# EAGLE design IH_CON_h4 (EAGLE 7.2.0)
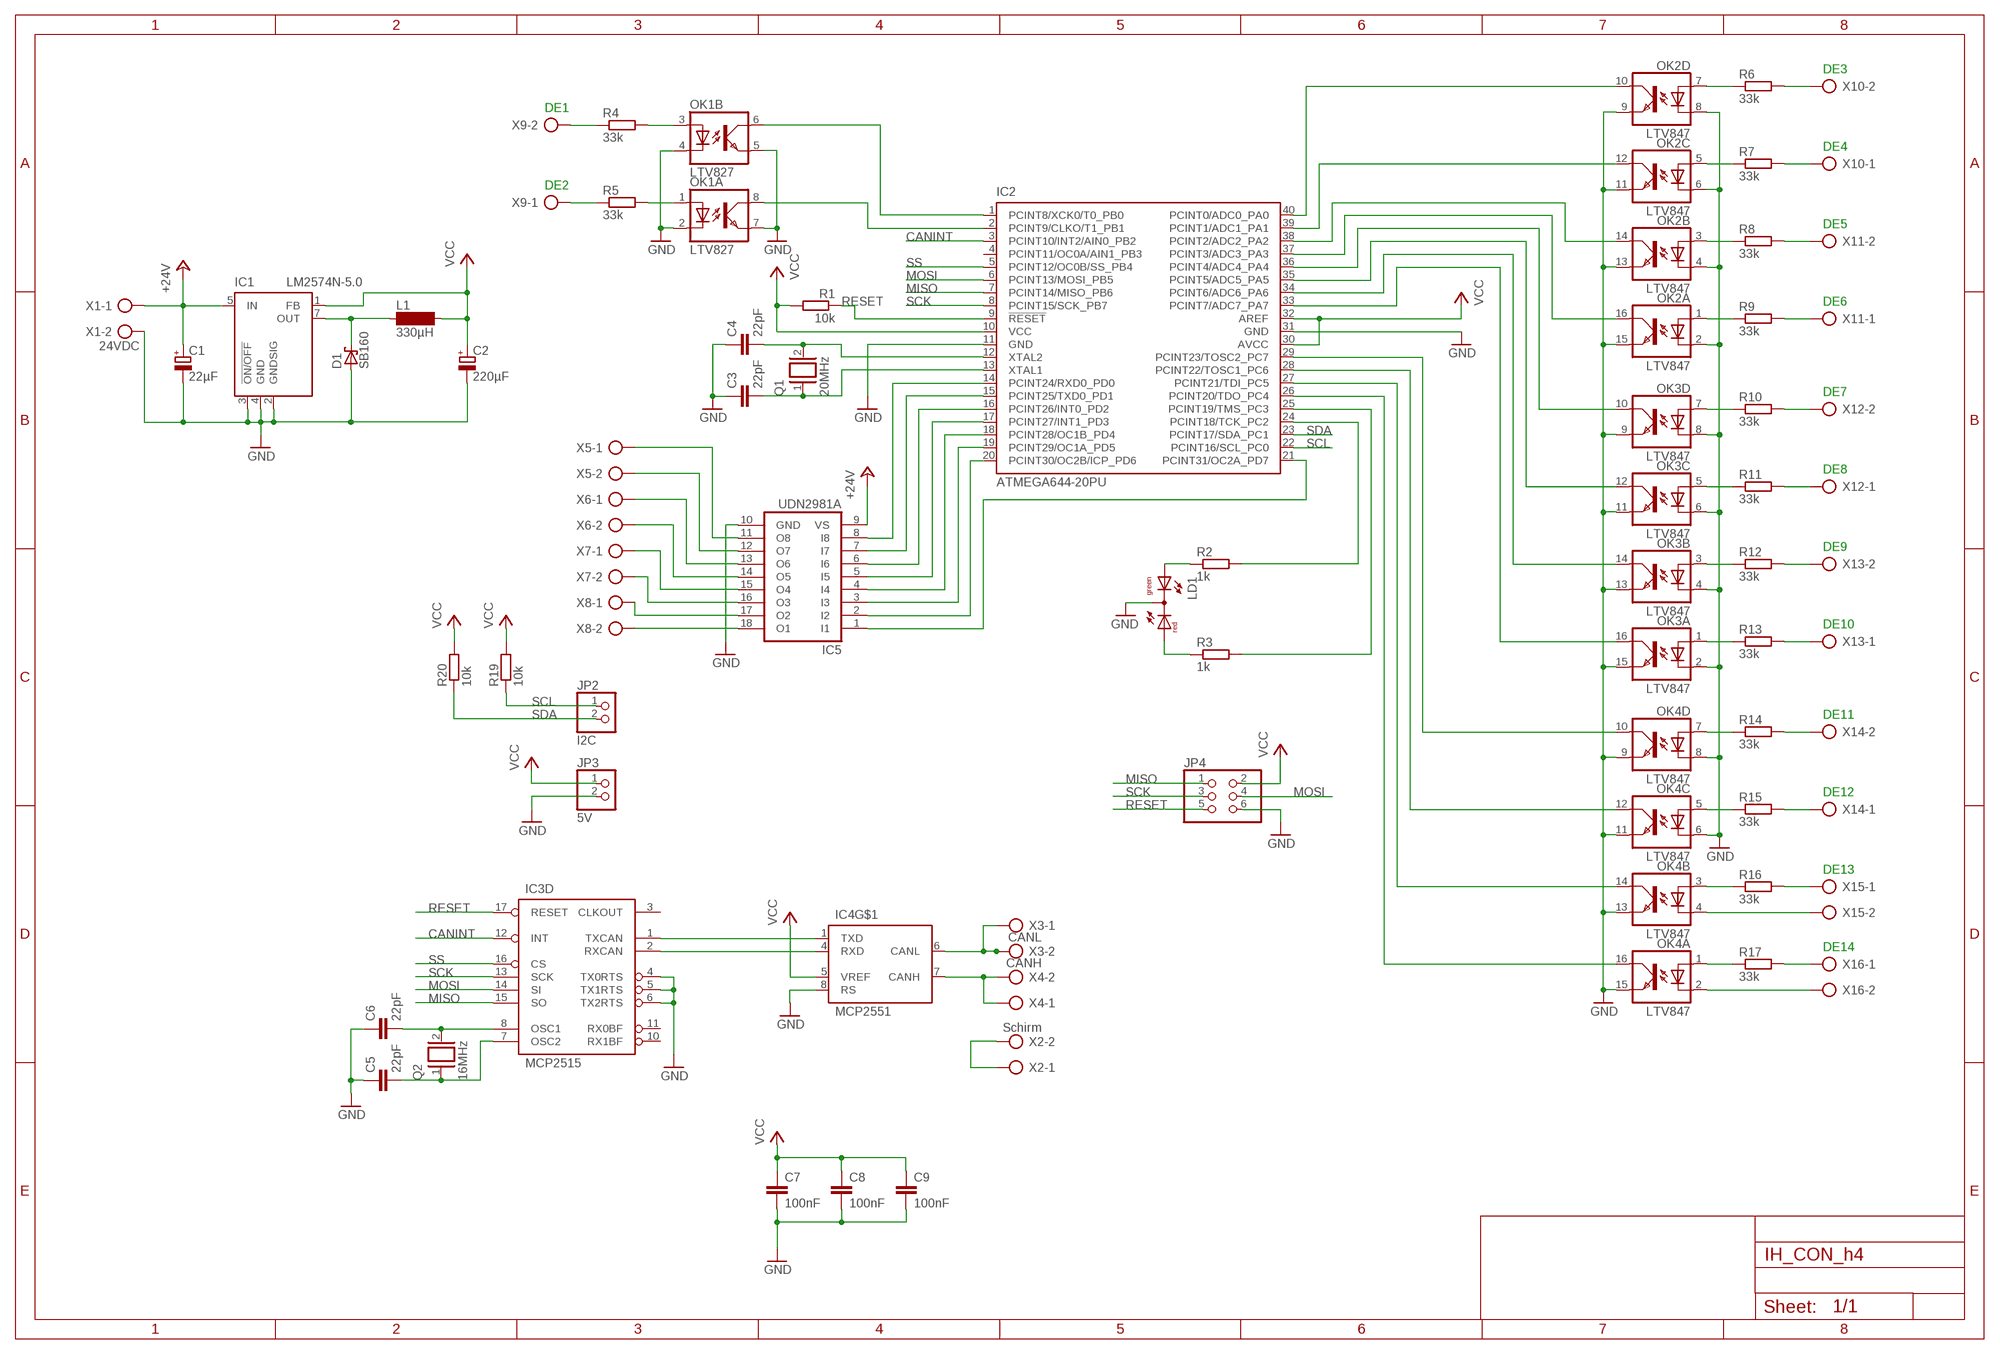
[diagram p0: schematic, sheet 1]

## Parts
C1  22µF  CPOL-EUE2-5  [E2-5]
C2  220µF  CPOL-EUE3.5-8  [E3,5-8]
C3  22pF  C-EUC0805  [C0805]
C4  22pF  C-EUC0805  [C0805]
C5  22pF  C-EUC0805  [C0805]
C6  22pF  C-EUC0805  [C0805]
C7  100nF  C-EUC0805  [C0805]
C8  100nF  C-EUC0805  [C0805]
C9  100nF  C-EUC0805  [C0805]
D1  SB160  SCHOTTKY-DIODEF126Z12  [F126Z12]
IC1  LM2574N-5.0  [DIL08]
IC2  ATMEGA644-20PU  [DIL40]
IC3  MCP2515  MCP2515P  [DIL18]
IC4  MCP2551  MCP2551DIL8  [DIL08]
IC5  UDN2981A  [DIL18]
JP2  I2C  PINHD-1X2  [1X02]
JP3  5V  PINHD-1X2  [1X02]
JP4  PINHD-2X3  [2X03]
L1  330µH  SD12-1000  [SD12_1000]
LD1  DUOLED-RG-C  [DUOLED-C-5MM]
OK1  LTV827  PC827  [DIL08]
OK2  LTV847  PC847  [DIL16]
OK3  LTV847  PC847  [DIL16]
OK4  LTV847  PC847  [DIL16]
Q1  20MHz  XTAL/S  [QS]
Q2  16MHz  XTAL/S  [QS]
R1  10k  R-EU_M0805  [M0805]
R2  1k  R-EU_M0805  [M0805]
R3  1k  R-EU_M0805  [M0805]
R4  33k  R-EU_0207/2V  [0207/2V]
R5  33k  R-EU_0207/2V  [0207/2V]
R6  33k  R-EU_0207/2V  [0207/2V]
R7  33k  R-EU_0207/2V  [0207/2V]
R8  33k  R-EU_0207/2V  [0207/2V]
R9  33k  R-EU_0207/2V  [0207/2V]
R10  33k  R-EU_0207/2V  [0207/2V]
R11  33k  R-EU_0207/2V  [0207/2V]
R12  33k  R-EU_0207/2V  [0207/2V]
R13  33k  R-EU_0207/2V  [0207/2V]
R14  33k  R-EU_0207/2V  [0207/2V]
R15  33k  R-EU_0207/2V  [0207/2V]
R16  33k  R-EU_0207/2V  [0207/2V]
R17  33k  R-EU_0207/2V  [0207/2V]
R19  10k  R-EU_M0805  [M0805]
R20  10k  R-EU_M0805  [M0805]
X1  24VDC  AK300/2  [AK300/2]
X2  Schirm  AK300/2  [AK300/2]
X3  CANL  AK300/2  [AK300/2]
X4  CANH  AK300/2  [AK300/2]
X5  AK300/2  [AK300/2]
X6  AK300/2  [AK300/2]
X7  AK300/2  [AK300/2]
X8  AK300/2  [AK300/2]
X9  AK300/2  [AK300/2]
X10  AK300/2  [AK300/2]
X11  AK300/2  [AK300/2]
X12  AK300/2  [AK300/2]
X13  AK300/2  [AK300/2]
X14  AK300/2  [AK300/2]
X15  AK300/2  [AK300/2]
X16  AK300/2  [AK300/2]

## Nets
+24V: C1.+ IC1.5(IN) IC5.9(VS) X1.1
CANINT: IC2.3(PCINT10/INT2/AIN0_PB2) IC3.12(D:INT)
GND: C1.- C2.- C3.1 C4.1 C5.1 C6.1 C7.2 C8.2 C9.2 D1.A IC1.2(GNDSIG) IC1.3(!ON/OFF) IC1.4(GND) IC2.11(GND) IC2.31(GND) IC3.4(D:TX0RTS) IC3.5(D:TX1RTS) IC3.6(D:TX2RTS) IC4.8(RS) IC5.10(GND) JP3.2 JP4.6 LD1.C OK1.2(A:C) OK1.4(B:C) OK1.5(B:EMIT) OK1.7(A:EMIT) OK2.2(A:C) OK2.4(B:C) OK2.6(C:C) OK2.8(D:C) OK2.9(D:EMIT) OK2.11(C:EMIT) OK2.13(B:EMIT) OK2.15(A:EMIT) OK3.2(A:C) OK3.4(B:C) OK3.6(C:C) OK3.8(D:C) OK3.9(D:EMIT) OK3.11(C:EMIT) OK3.13(B:EMIT) OK3.15(A:EMIT) OK4.6(C:C) OK4.8(D:C) OK4.9(D:EMIT) OK4.11(C:EMIT) OK4.13(B:EMIT) OK4.15(A:EMIT) X1.2
MISO: IC2.7(PCINT14/MISO_PB6) IC3.15(D:SO) JP4.1
MOSI: IC2.6(PCINT13/MOSI_PB5) IC3.14(D:SI) JP4.4
N$1: IC3.1(D:TXCAN) IC4.1(TXD)
N$2: IC3.2(D:RXCAN) IC4.4(RXD)
N$3: C6.2 IC3.8(D:OSC1) Q2.2
N$4: C5.2 IC3.7(D:OSC2) Q2.1
N$5: IC2.14(PCINT24/RXD0_PD0) IC5.8(I8)
N$6: IC2.15(PCINT25/TXD0_PD1) IC5.7(I7)
N$7: C4.2 IC2.12(XTAL2) Q1.2
N$8: C3.2 IC2.13(XTAL1) Q1.1
N$9: IC2.21(PCINT31/OC2A_PD7) IC5.1(I1)
N$10: IC2.16(PCINT26/INT0_PD2) IC5.6(I6)
N$11: IC2.17(PCINT27/INT1_PD3) IC5.5(I5)
N$12: IC2.18(PCINT28/OC1B_PD4) IC5.4(I4)
N$13: IC2.19(PCINT29/OC1A_PD5) IC5.3(I3)
N$14: IC2.20(PCINT30/OC2B/ICP_PD6) IC5.2(I2)
N$16: IC4.6(CANL) X3.1 X3.2
N$17: IC4.7(CANH) X4.1 X4.2
N$18: IC5.18(O1) X8.2
N$19: IC5.17(O2) X8.1
N$20: IC5.16(O3) X7.2
N$21: IC5.15(O4) X7.1
N$22: IC5.14(O5) X6.2
N$23: IC5.13(O6) X6.1
N$24: IC5.12(O7) X5.2
N$25: IC5.11(O8) X5.1
N$26: IC2.25(PCINT19/TMS_PC3) R3.2
N$27: R6.2 X10.2
N$28: OK4.1(A:A) R17.1
N$29: OK4.3(B:A) R16.1
N$30: OK4.5(C:A) R15.1
N$31: OK4.7(D:A) R14.1
N$32: OK3.1(A:A) R13.1
N$33: IC2.24(PCINT18/TCK_PC2) R2.2
N$34: OK3.3(B:A) R12.1
N$35: OK3.5(C:A) R11.1
N$36: OK3.7(D:A) R10.1
N$37: OK2.1(A:A) R9.1
N$38: OK2.3(B:A) R8.1
N$39: OK2.5(C:A) R7.1
N$40: OK2.7(D:A) R6.1
N$41: R7.2 X10.1
N$42: LD1.AX(AG) R2.1
N$43: LD1.AR R3.1
N$45: R8.2 X11.2
N$46: R9.2 X11.1
N$47: R10.2 X12.2
N$48: R11.2 X12.1
N$49: R12.2 X13.2
N$50: R13.2 X13.1
N$51: R14.2 X14.2
N$52: R15.2 X14.1
N$53: R16.2 X15.1
N$54: X2.1 X2.2
N$55: R17.2 X16.1
N$56: OK4.2(A:C) X16.2
N$57: IC2.33(PCINT7/ADC7_PA7) OK3.16(A:COL)
N$58: IC2.34(PCINT6/ADC6_PA6) OK3.14(B:COL)
N$59: IC2.35(PCINT5/ADC5_PA5) OK3.12(C:COL)
N$60: IC2.36(PCINT4/ADC4_PA4) OK3.10(D:COL)
N$61: IC2.37(PCINT3/ADC3_PA3) OK2.16(A:COL)
N$62: IC2.38(PCINT2/ADC2_PA2) OK2.14(B:COL)
N$63: IC2.39(PCINT1/ADC1_PA1) OK2.12(C:COL)
N$64: IC2.40(PCINT0/ADC0_PA0) OK2.10(D:COL)
N$65: IC2.29(PCINT23/TOSC2_PC7) OK4.10(D:COL)
N$66: IC2.28(PCINT22/TOSC1_PC6) OK4.12(C:COL)
N$67: IC2.27(PCINT21/TDI_PC5) OK4.14(B:COL)
N$68: IC2.26(PCINT20/TDO_PC4) OK4.16(A:COL)
N$71: OK1.3(B:A) R4.2
N$72: R5.1 X9.1
N$73: R4.1 X9.2
N$74: IC2.2(PCINT9/CLKO/T1_PB1) OK1.8(A:COL)
N$75: IC2.1(PCINT8/XCK0/T0_PB0) OK1.6(B:COL)
N$76: D1.C IC1.7(OUT) L1.1
N$100: OK4.4(B:C) X15.2
OK1: OK1.1(A:A) R5.2
RESET: IC2.9(!RESET) IC3.17(D:RESET) JP4.5 R1.1
SCK: IC2.8(PCINT15/SCK_PB7) IC3.13(D:SCK) JP4.3
SCL: IC2.22(PCINT16/SCL_PC0) JP2.1 R19.1
SDA: IC2.23(PCINT17/SDA_PC1) JP2.2 R20.1
SS: IC2.5(PCINT12/OC0B/SS_PB4) IC3.16(D:CS)
VCC: C2.+ C7.1 C8.1 C9.1 IC1.1(FB) IC2.10(VCC) IC2.30(AVCC) IC2.32(AREF) IC4.5(VREF) JP3.1 JP4.2 L1.2 R1.2 R19.2 R20.2
Unconnected: IC2.4(PCINT11/OC0A/AIN1_PB3) IC3.3(D:CLKOUT) IC3.10(D:RX1BF) IC3.11(D:RX0BF)

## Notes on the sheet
- DE3
- DE1
- DE4
- DE2
- DE5
- DE6
- DE7
- DE8
- DE9
- DE10
- DE11
- DE12
- DE13
- DE14

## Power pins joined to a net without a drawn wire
GND: IC3.9(P:GND) IC4.2(GND)
VCC: IC3.18(P:VCC) IC4.3(VCC)

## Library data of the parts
C1 C2 = rcl:CPOL-EU: POLARIZED CAPACITOR, European symbol
C3-C9 = rcl:C-EU: CAPACITOR, European symbol
D1 = diode:SCHOTTKY-DIODE: Schottky Diode
IC1 = linear:LM2574?-*: SIMPLE SWITCHER 0.5A Step-Down Voltage Regulator Source: http://cache.national.com/ds/LM/LM2574.pdf
IC2 = atmel:ATMEGA644-*PU: 8-bit Microcontroller with 64K Bytes In-System Programmable Flash Auto generated by make-symbol-device-package-bsdl.ulp Rev. 34 Source: http://www.atmel.com/dyn/resources/prod_documents/doc2593.pdf; MPN: ATMEGA644-20PU; OC_FARNELL: 1288340; OC_NEWARK: 23M5060
IC3 = can:MCP2515: MC2515 Stand-Alone CAN Controller With SPI Interface, Microchip
IC4 = can:MCP2551: CAN Tranceiver Microchip
IC5 = uln-udn:UDN298*: DRIVER ARRAY Source: Allegro Microsystems Inc. / UDN2981-UDN2984.pdf
JP2 JP3 = pinhead:PINHD-1X2: PIN HEADER
JP4 = pinhead:PINHD-2X3: PIN HEADER
L1 = inductor-neosid:SD12: INDUCTOR; OC_FARNELL: unknown; OC_NEWARK: unknown
LD1 = led:DUOLED-RG-C: DUO LED 2 colors (red/green), 5 mm, round, common Cathode www.ligitek.com or other producers.
OK1 = optocoupler:PC827: SHARP OPTO COUPLER; OC_FARNELL: unknown; OC_NEWARK: unknown
OK2-OK4 = optocoupler:PC847: SHARP OPTO COUPLER; OC_FARNELL: 9707735; OC_NEWARK: unknown
Q1 Q2 = special:XTAL/S: CRYSTAL
R1 = rcl:R-EU_: RESISTOR, European symbol
R2-R17 R19 R20 = resistor:R-EU_: RESISTOR, European symbol
X1-X16 = con-ptr500:AK300/2: CONNECTOR; OC_FARNELL: unknown; OC_NEWARK: unknown

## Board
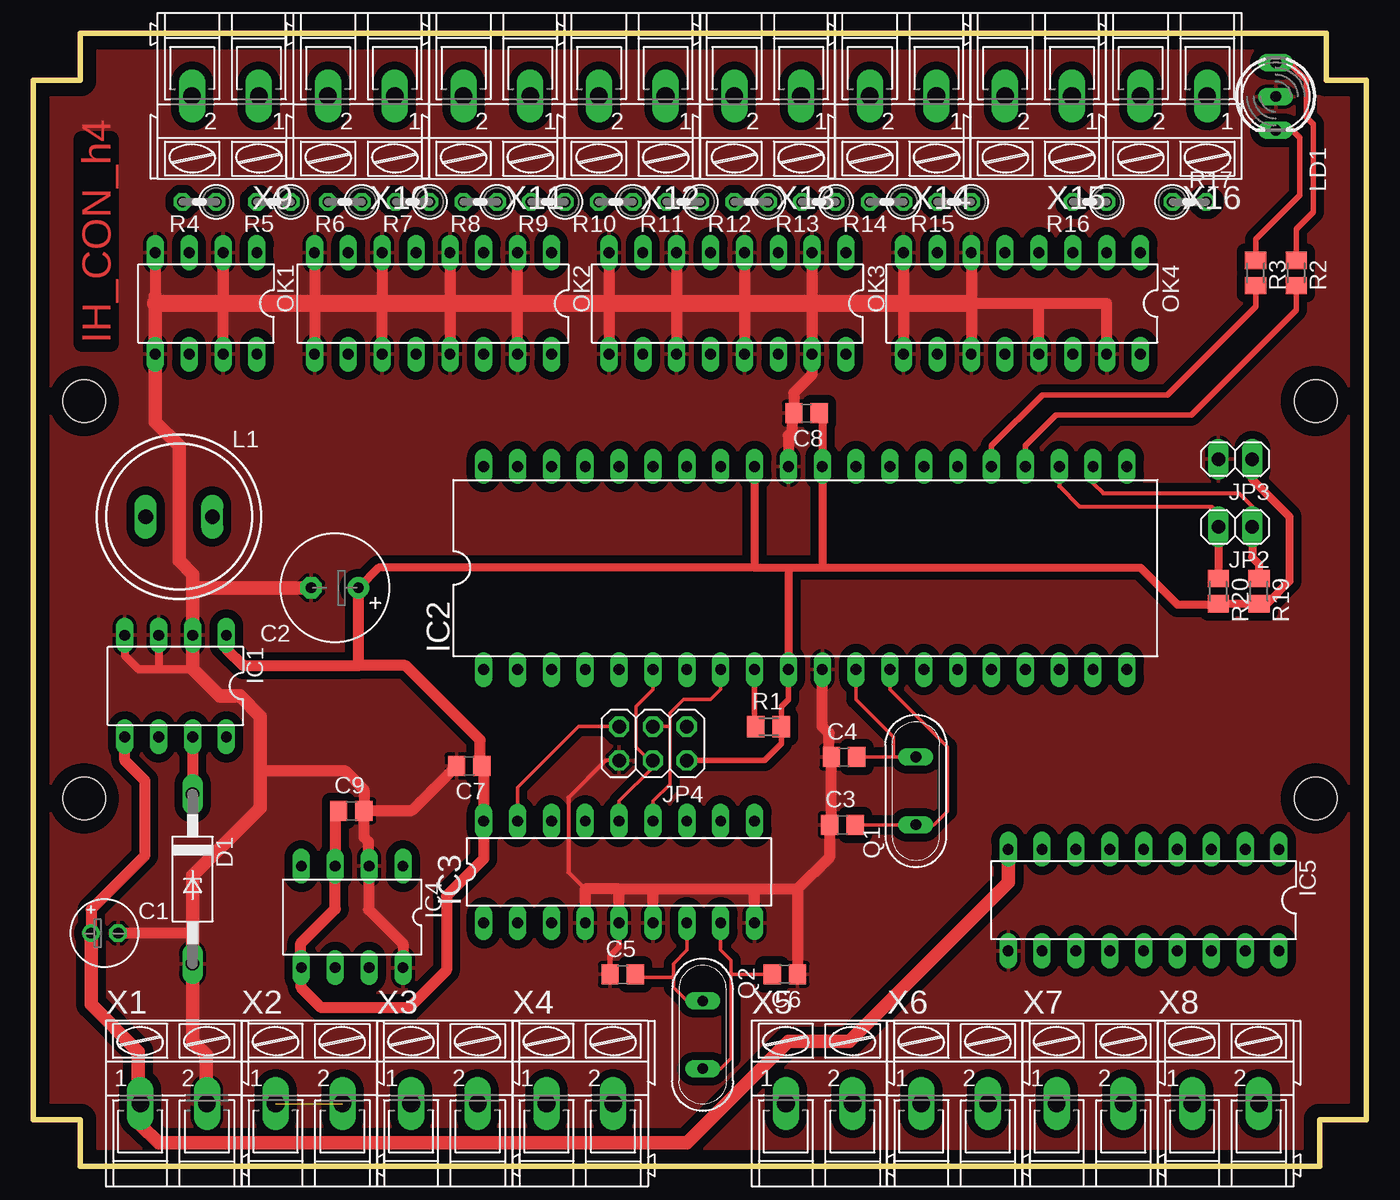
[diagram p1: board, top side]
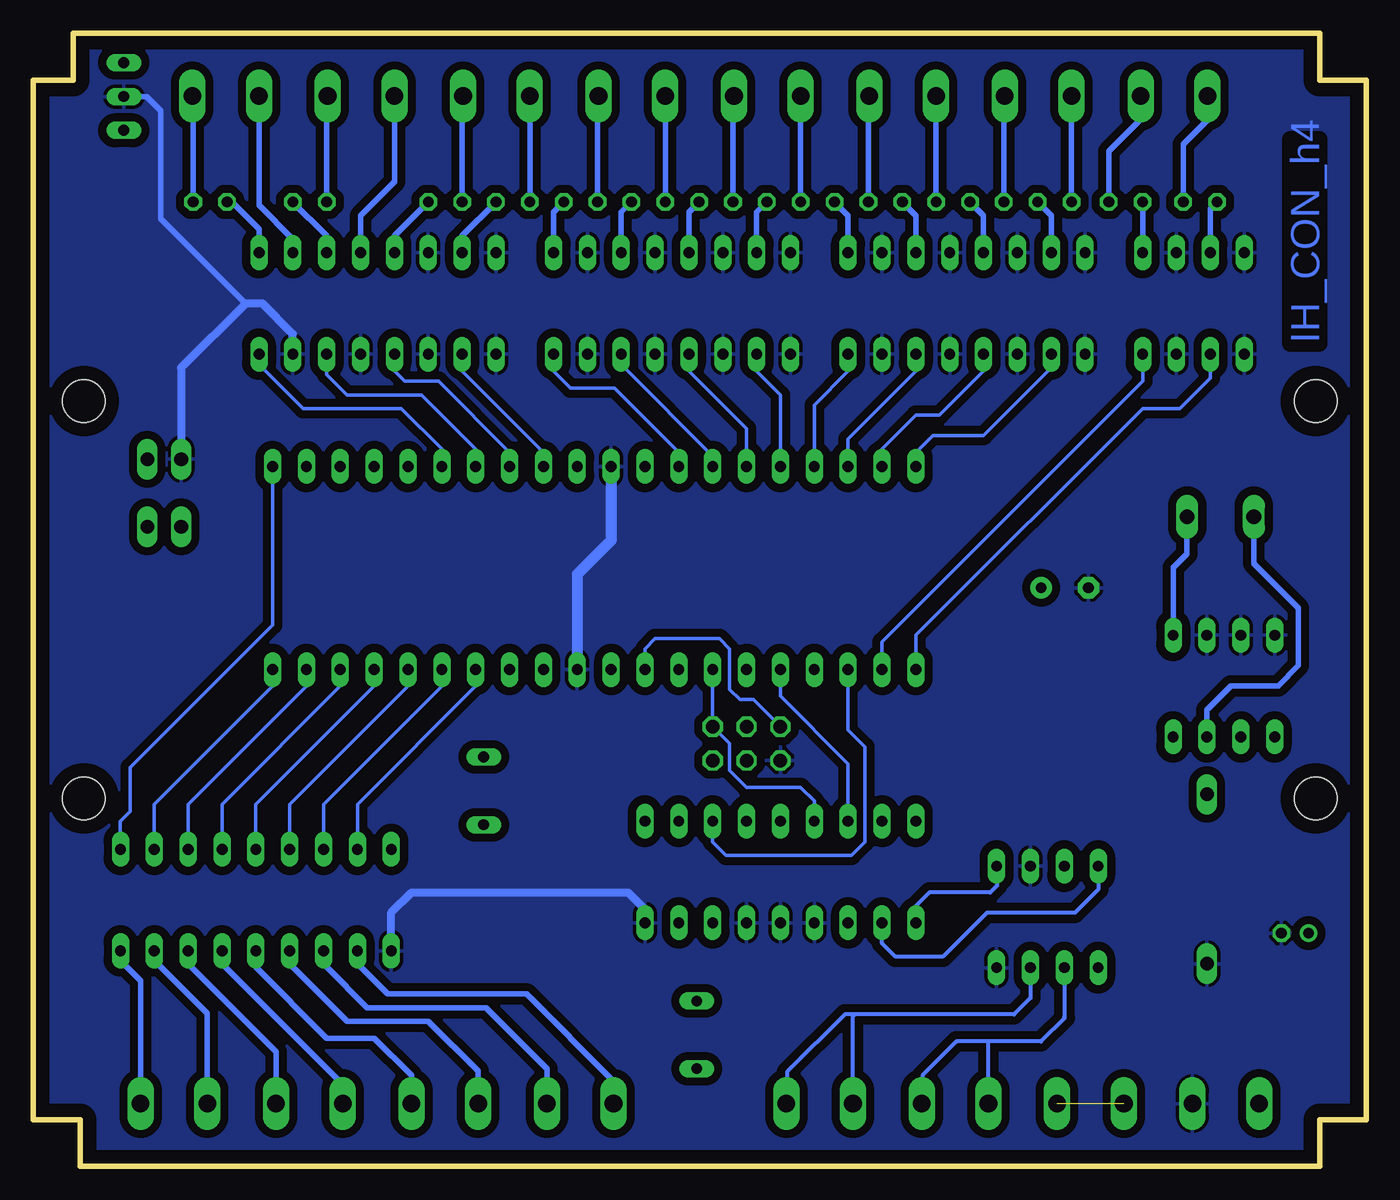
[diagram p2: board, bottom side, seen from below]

Size 100 x 85 mm. Coordinates in mm from the lower left corner, seen from the top.
Outline: 100,3.5 100,80
Outline: 100,3.5 100,81.5 97,81.5 97,85 3.5,85 3.5,81.5 0,81.5 0,3.5 3.5,3.5 3.5,0 96.5,0 96.5,3.5 100,3.5
Copper layers (1*16): Top 0.035mm / dielectric 1.5mm / Bottom 0.035mm
Design rules "default *": minimum track width 10mil, minimum drill 36mil, track to track 15mil, track to pad 15mil, pad to pad 10mil, via to via 10mil, smd to smd 10mil, copper to edge 40mil, drill to drill 8mil, minimum pad ring 10mil, minimum via ring 8mil, stop-mask expansion 4mil, vias tented up to drill 0mil, thermal gap 10mil
Holes 3.2 mm at 3.8,27.6 3.8,57.4 96.2,27.6 96.2,57.4

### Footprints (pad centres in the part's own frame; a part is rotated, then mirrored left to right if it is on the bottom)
E2-5 = drill 0.813 pad 1.27: + -1.016,0 | drill 0.813 pad 1.27 octagon: - 1.016,0
E3,5-8 = drill 0.813 pad 1.6: + -1.778,0 | drill 0.813 pad 1.6 octagon: - 1.778,0
C0805 = smd 1.3 x 1.5: 1 -0.95,0; 2 0.95,0
F126Z12 = drill 1.016 long: A 6.35,0; C -6.35,0
DIL08 = drill 0.813 pad 1.27 long: 1 -3.81,-3.81; 2 -1.27,-3.81; 3 1.27,-3.81; 4 3.81,-3.81; 5 3.81,3.81; 6 1.27,3.81; 7 -1.27,3.81; 8 -3.81,3.81
DIL40 = drill 0.813 long: 1 -24.13,-7.62; 2 -21.59,-7.62; 3 -19.05,-7.62; 4 -16.51,-7.62; 5 -13.97,-7.62; 6 -11.43,-7.62; 7 -8.89,-7.62; 8 -6.35,-7.62; 9 -3.81,-7.62; 10 -1.27,-7.62; 11 1.27,-7.62; 12 3.81,-7.62; 13 6.35,-7.62; 14 8.89,-7.62; 15 11.43,-7.62; 16 13.97,-7.62; 17 16.51,-7.62; 18 19.05,-7.62; 19 21.59,-7.62; 20 24.13,-7.62; 21 24.13,7.62; 22 21.59,7.62; 23 19.05,7.62; 24 16.51,7.62; 25 13.97,7.62; 26 11.43,7.62; 27 8.89,7.62; 28 6.35,7.62; 29 3.81,7.62; 30 1.27,7.62; 31 -1.27,7.62; 32 -3.81,7.62; 33 -6.35,7.62; 34 -8.89,7.62; 35 -11.43,7.62; 36 -13.97,7.62; 37 -16.51,7.62; 38 -19.05,7.62; 39 -21.59,7.62; 40 -24.13,7.62
DIL18 = drill 0.813 long: 1 -10.16,-3.81; 2 -7.62,-3.81; 3 -5.08,-3.81; 4 -2.54,-3.81; 5 0,-3.81; 6 2.54,-3.81; 7 5.08,-3.81; 8 7.62,-3.81; 9 10.16,-3.81; 10 10.16,3.81; 11 7.62,3.81; 12 5.08,3.81; 13 2.54,3.81; 14 0,3.81; 15 -2.54,3.81; 16 -5.08,3.81; 17 -7.62,3.81; 18 -10.16,3.81
DIL08' = drill 0.813 long: 1 -3.81,-3.81; 2 -1.27,-3.81; 3 1.27,-3.81; 4 3.81,-3.81; 5 3.81,3.81; 6 1.27,3.81; 7 -1.27,3.81; 8 -3.81,3.81
1X02 = drill 1.016 long: 1 -1.27,0; 2 1.27,0
2X03 = drill 1.016 octagon: 1 -2.54,-1.27; 2 -2.54,1.27; 3 0,-1.27; 4 0,1.27; 5 2.54,-1.27; 6 2.54,1.27
SD12_1000 = drill 1.1 long: 1 -2.5,0; 2 2.5,0
DUOLED-C-5MM = drill 0.813 long: AR 2.54,0; AX -2.54,0; C 0,0
DIL16 = drill 0.813 long: 1 -8.89,-3.81; 2 -6.35,-3.81; 3 -3.81,-3.81; 4 -1.27,-3.81; 5 1.27,-3.81; 6 3.81,-3.81; 7 6.35,-3.81; 8 8.89,-3.81; 9 8.89,3.81; 10 6.35,3.81; 11 3.81,3.81; 12 1.27,3.81; 13 -1.27,3.81; 14 -3.81,3.81; 15 -6.35,3.81; 16 -8.89,3.81
QS = drill 0.8 long: 1 -2.54,0; 2 2.54,0
M0805 = smd 1.3 x 1.6: 1 -0.95,0; 2 0.95,0
0207/2V = drill 0.813 octagon: 1 -1.27,0; 2 1.27,0
AK300/2 = drill 1.321 long: 1 -2.515,0; 2 2.489,0

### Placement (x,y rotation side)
C1  5.34,17.49 0 top
C2  22.61,43.39 180 top
C3  60.7,25.61 0 top
C4  60.83,30.69 0 top
C5  44.22,14.38 0 top
C6  56.38,14.41 180 top
C7  32.7,30.03 180 top
C8  58.02,56.5 180 top
C9  23.86,26.66 0 top
D1  11.95,21.55 270 top
IC1  10.68,36.03 180 top
IC2  57.92,44.88 0 top
IC3  43.95,22.08 0 top
IC4  MCP2551  [DIL08']  23.92,18.71 180 top
IC5  83.3,19.96 180 top
JP2  90.18,47.97 180 top
JP3  90.18,53.05 180 top
JP4  46.49,31.71 180 top
L1  10.93,48.73 0 top
LD1  93.21,80.26 270 top
OK1  LTV827  [DIL08']  12.96,64.73 180 top
OK2  29.98,64.73 180 top
OK3  52.08,64.73 180 top
OK4  74.18,64.73 180 top
Q1  66.21,28.16 90 top
Q2  50.21,9.85 270 top
R1  55.16,32.97 0 top
R2  94.75,67.02 270 top
R3  91.7,67.02 270 top
R4  12.45,72.35 180 top
R5  18.04,72.35 180 top
R6  23.38,72.35 180 top
R7  28.46,72.35 180 top
R8  33.54,72.35 180 top
R9  38.62,72.35 180 top
R10  43.7,72.35 180 top
R11  48.78,72.35 180 top
R12  53.86,72.35 180 top
R13  58.94,72.35 180 top
R14  64.02,72.35 180 top
R15  69.1,72.35 180 top
R16  79.26,72.35 180 top
R17  86.73,72.35 0 top
R19  91.96,43.14 270 top
R20  88.91,43.14 270 top
X1  10.54,4.7 0 top
X2  20.7,4.7 0 top
X3  30.86,4.7 0 top
X4  41.02,4.7 0 top
X5  58.98,4.7 0 top
X6  69.14,4.7 0 top
X7  79.3,4.7 0 top
X8  89.46,4.7 0 top
X9  14.4,80.3 180 top
X10  24.6,80.3 180 top
X11  34.76,80.3 180 top
X12  44.92,80.3 180 top
X13  55.08,80.3 180 top
X14  65.24,80.3 180 top
X15  75.4,80.3 180 top
X16  85.56,80.3 180 top

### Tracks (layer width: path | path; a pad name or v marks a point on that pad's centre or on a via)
+24V
  Top 0.813: C1.+ 4.33,19.26 8.39,23.33 8.39,28.92 6.87,30.44 IC1.5
  Top 1.016: IC5.9 73.16,23.76 73.16,21.3 61.22,9.36 56.65,9.36 49.03,1.74 9.41,1.74 8.03,3.12 X1.1 7.88,4.84 7.88,8.6 4.33,12.15 C1.+
CANINT
  Bottom 0.254: IC2.3 38.87,32.73 37.6,31.46 37.6,24.34 38.62,23.33 48.01,23.33 49.03,24.34 IC3.12
GND
  Top 0.305: JP4.6 42.93,30.44 40.14,27.65 40.14,22.06 41.41,20.79
  Top 0.406: C5.1 43.27,15.79 43.95,16.47 IC3.5
  Top 0.61: IC1.4 6.87,38.31 7.88,37.3 9.41,37.3 | 9.41,37.3 11.95,37.3 | IC1.3 9.41,37.3
  Top 0.813: OK1.4 9.15,65.24 9.15,64.73 | OK1.7 OK1.2 14.23,64.73 13.98,64.73 | OK2.9 21.09,64.73 OK2.8 | OK2.11 26.17,64.73 OK2.6 | OK2.15 36.33,64.73 OK2.2 | OK2.13 31.25,64.73 OK2.4 | OK3.11 48.27,64.73 OK3.6 | OK3.9 43.19,64.73 OK3.8 | OK3.13 53.35,64.73 OK3.4 | OK4.9 OK4.8 65.29,64.73 65.54,64.73 | OK4.6 70.37,64.73 | 70.37,64.73 OK4.11 | OK4.13 75.45,64.73 | 75.45,64.73 70.37,64.73 | OK4.15 80.53,64.73 75.45,64.73 | OK3.2 58.43,64.73 OK3.15 58.43,59.4 57.07,58.04 C8.2 56.9,56.34 56.9,55.08 56.65,54.82 IC2.31 | C1.- 11.95,17.49 11.95,15.96 D1.A | C7.2 28.38,26.66 C9.2 | C9.2 24.81,24.69 25.15,24.34 25.15,22.55 IC4.2 25.15,22.48 25.15,19.26 27.73,16.69 IC4.8 | 17.03,29.68 23.38,29.68 24.81,28.24 C9.2 | IC2.11 59.19,32.98 59.7,32.47 59.7,31.12 C4.1 59.88,25.73 C3.1 59.75,23.21 57.33,20.79 | IC3.9 54.11,20.79 | 54.11,20.79 57.33,20.79 | 57.33,20.79 C6.1 | IC3.6 46.49,20.79 | 46.49,20.79 54.11,20.79 | IC3.5 43.95,20.79 | 43.95,20.79 46.49,20.79 | 43.95,20.79 41.41,20.79 IC3.4
  Top 1.016: X1.2 12.96,4.77 12.96,8.34 11.95,9.36 D1.A | 11.95,15.96 11.95,21.8 17.03,26.88 17.03,29.68 17.03,33.74 15.5,35.27 13.98,35.27 11.95,37.3 IC1.2 11.95,43.39 | 11.95,43.39 11.95,44.41 10.93,45.43 10.93,54.06 9.15,55.84 OK1.5 9.15,65.24 | C2.- 11.95,43.39
  Top 1.27: 70.37,64.73 65.54,64.73 58.43,64.73 53.35,64.73 48.27,64.73 43.19,64.73 36.33,64.73 31.25,64.73 26.17,64.73 21.09,64.73 13.98,64.73 9.15,64.73
  Bottom 0.406: LD1.C 91.48,80.26 90.43,79.21 90.43,71.08 84.08,64.73
  Bottom 0.61: OK4.15 80.53,62.44 82.81,64.73 84.08,64.73 88.91,59.9 JP3.2 | IC5.10 73.14,19.03 71.64,20.53 55.38,20.53 54.11,19.26 IC3.9
  Bottom 0.813: IC2.31 56.65,46.95 59.19,44.41 IC2.11
  pour Bottom (isolate 0.61): -5.33,89.88 103.39,89.88 103.39,-4.1 -5.07,-4.1 -5.07,87.34
  pour Top (isolate 0.61): -7.1,90.64 105.67,90.64 105.67,-6.14 -7.1,-6.14 -7.1,86.83
MISO
  Bottom 0.254: IC2.7 JP4.1 47.76,31.71 47.76,29.68 46.49,28.41 42.43,28.41 41.41,27.39 IC3.15
MOSI
  Top 0.254: IC3.14 43.95,27.39 46.49,29.93 JP4.4 46.24,30.44 45.22,31.46 45.22,34.5 46.49,35.77 IC2.6
N$1
  Bottom 0.305: IC4.1 27.69,22.52 27.69,21.04 28.2,20.53 32.77,20.53 33.79,19.52 IC3.1
N$2
  Bottom 0.305: IC4.4 20.11,20.75 21.85,19.01 28.46,19.01 31.76,15.71 35.31,15.71 36.33,16.72 IC3.2
N$3
  Top 0.254: Q2.2 51.56,7.31 52.33,8.09 52.33,14.44 | 52.33,14.44 52.33,15.45 51.57,16.22 IC3.8 | C6.2 52.36,14.41 52.33,14.44
N$4
  Top 0.254: Q2.1 49.04,12.39 48.01,13.42 48.01,14.18 | 48.01,14.18 48.01,15.2 49.03,16.22 IC3.7 | C5.2 45.37,14.18 48.01,14.18
N$5
  Bottom 0.254: IC2.14 66.81,36.03 75.68,27.16 IC5.8
N$6
  Bottom 0.254: IC2.15 69.35,36.03 78.22,27.16 IC5.7
N$7
  Top 0.254: C4.2 63.77,30.69 64.02,30.69 64.52,30.69 | 64.52,30.69 Q1.2 | IC2.12 61.73,35.01 64.52,32.22 64.52,30.69
N$8
  Top 0.254: C3.2 Q1.1 66.22,25.61 67.57,25.61 68.59,26.63 68.59,31.46 64.27,35.77 IC2.13
N$9
  Bottom 0.254: IC2.21 82.05,40.6 92.72,29.93 92.72,26.63 93.48,25.87 93.48,23.79 IC5.1
N$10
  Bottom 0.254: IC2.16 71.89,36.03 80.76,27.16 IC5.6
N$11
  Bottom 0.254: IC2.17 74.43,36.03 83.3,27.16 IC5.5
N$12
  Bottom 0.254: IC2.18 76.97,36.03 85.84,27.16 IC5.4
N$13
  Bottom 0.254: IC2.19 79.51,36.03 88.38,27.16 IC5.3
N$14
  Bottom 0.254: IC2.20 82.05,36.03 90.92,27.16 IC5.2
N$16
  Bottom 0.305: IC4.6 22.65,11.17 22.61,11.14 24.39,9.36 28.46,9.36 | 28.46,9.36 30.74,9.36 33.28,6.82 33.28,4.77 X3.2 | X3.1 28.34,9.25 28.46,9.36
N$17
  Bottom 0.305: IC4.7 25.19,12.63 26.42,11.39 38.36,11.39 | 38.36,11.39 39.12,11.39 43.44,7.07 43.44,4.77 X4.2 | X4.1 38.51,11.25 38.36,11.39
N$18
  Bottom 0.406: IC5.18 93.23,15.92 93.23,15.2 91.95,13.92 X8.2
N$19
  Bottom 0.406: IC5.17 90.69,15.92 90.69,15.2 86.94,11.46 X8.1
N$20
  Bottom 0.406: IC5.16 88.15,15.92 88.15,14.95 81.79,8.59 X7.2
N$21
  Bottom 0.406: IC5.15 85.61,15.92 85.61,14.95 76.78,6.12 X7.1
N$22
  Bottom 0.406: IC5.14 83.32,16.14 83.32,14.95 77.99,9.61 74.43,9.61 71.63,6.81 X6.2
N$23
  Bottom 0.406: IC5.13 80.53,15.92 80.53,14.95 76.46,10.88 70.37,10.88 66.62,7.14 X6.1
N$24
  Bottom 0.406: IC5.12 77.99,15.92 77.99,14.95 74.94,11.9 66.05,11.9 61.47,7.32 X5.2
N$25
  Bottom 0.406: IC5.11 75.45,15.92 75.45,14.95 73.41,12.91 63,12.91 56.47,6.38 X5.1
N$26
  Top 0.406: R3.2 91.7,64.48 85.1,57.87 75.7,57.87 71.89,54.06 IC2.25
N$27
  Bottom 0.406: X10.2 R6.2
N$28
  Bottom 0.406: OK4.1 83.07,70.32 85.1,72.35 R17.1
N$29
  Bottom 0.406: R16.1 77.99,69.81 OK4.3
N$30
  Bottom 0.406: R15.1 72.91,69.81 OK4.5
N$31
  Bottom 0.406: R14.1 67.83,69.81 OK4.7
N$32
  Bottom 0.406: R13.1 60.97,71.59 OK3.1
N$33
  Top 0.406: IC2.24 74.43,54.06 76.72,56.35 86.88,56.35 94.75,64.22 R2.2
N$34
  Bottom 0.406: R12.1 55.89,71.59 OK3.3
N$35
  Bottom 0.406: R11.1 50.81,71.59 OK3.5
N$36
  Bottom 0.406: R10.1 45.73,71.59 OK3.7
N$37
  Bottom 0.406: R9.1 38.87,71.33 OK2.1
N$38
  Bottom 0.406: R8.1 33.79,71.33 OK2.3
N$39
  Bottom 0.406: R7.1 28.71,71.33 OK2.5
N$40
  Bottom 0.406: R6.1 23.63,71.33 OK2.7
N$41
  Bottom 0.406: X10.1 27.19,80.23 R7.2
N$42
  Top 0.406: R2.1 94.75,70.32 96.02,71.59 96.02,78.19 95.51,78.7 95.51,81.49 94.21,82.8 LD1.AX
N$43
  Top 0.406: LD1.AR 94.46,77.72 95,77.18 95,72.86 91.7,69.56 R3.1
N$45
  Bottom 0.406: X11.2 R8.2
N$46
  Bottom 0.406: X11.1 37.35,80.23 R9.2
N$47
  Bottom 0.406: X12.2 R10.2
N$48
  Bottom 0.406: X12.1 47.51,80.23 R11.2
N$49
  Bottom 0.406: X13.2 R12.2
N$50
  Bottom 0.406: X13.1 57.67,80.23 R13.2
N$51
  Bottom 0.406: X14.2 R14.2
N$52
  Bottom 0.406: X14.1 67.83,80.23 R15.2
N$53
  Bottom 0.406: X15.1 77.99,80.23 R16.2
N$54  (1 unrouted)
N$55
  Bottom 0.406: X16.1 88,80.23 R17.2
N$56
  Bottom 0.406: X16.2 83.07,72.1 80.53,69.56 OK4.2
N$57
  Bottom 0.254: OK3.16 60.97,59.65 59.7,58.38 56.4,58.38 51.57,53.55 IC2.33
N$58
  Bottom 0.254: OK3.14 55.63,60.67 55.63,59.9 49.03,53.3 IC2.34
N$59
  Bottom 0.254: OK3.12 50.81,59.65 46.49,55.33 IC2.35
N$60
  Bottom 0.254: OK3.10 45.73,59.65 43.95,57.87 IC2.36
N$61
  Bottom 0.254: OK2.16 38.87,59.65 41.41,57.11 IC2.37
N$62
  Bottom 0.254: OK2.14 33.79,59.65 38.87,54.57 IC2.38
N$63
  Bottom 0.254: OK2.12 28.71,59.65 32.01,56.35 33.79,56.35 36.33,53.81 IC2.39
N$64
  Bottom 0.254: OK2.10 23.63,59.9 28.71,54.82 32.52,54.82 33.79,53.55 IC2.40
N$65
  Bottom 0.254: IC2.29 61.98,52.76 61.98,53.81 67.83,59.65 OK4.10
N$66
  Bottom 0.254: IC2.28 64.27,53.55 69.6,58.89 72.14,58.89 72.91,59.65 OK4.12
N$67
  Bottom 0.254: IC2.27 66.81,53.81 70.87,57.87 76.46,57.87 77.99,59.4 OK4.14
N$68
  Bottom 0.254: IC2.26 69.35,53.81 72.4,56.86 79.76,56.86 83.07,60.16 OK4.16
N$71
  Bottom 0.406: R4.2 11.69,71.84 OK1.3
N$72
  Bottom 0.406: X9.1 17.03,80.19 17.03,78.45 19.31,76.16 R5.1
N$73
  Bottom 0.406: X9.2 11.95,80.27 11.95,78.45 13.72,76.67 R4.1
N$74
  Bottom 0.254: OK1.8 16.77,58.89 36.33,39.33 IC2.2
N$75
  Bottom 0.254: OK1.6 11.69,59.14 13.98,56.86 16.77,56.86 33.79,39.84 IC2.1
N$76
  Top 0.813: IC1.7 D1.C
  Bottom 0.406: IC1.7 11.95,34.25 10.17,36.03 6.61,36.03 5.09,37.55 5.09,41.87 8.43,45.21 L1.1
N$100
  Bottom 0.406: X15.2 72.91,73.87 75.45,71.33 OK4.4
OK1
  Bottom 0.406: R5.2 OK1.1
RESET
  Top 0.254: IC3.17 36.33,28.41 40.9,32.98 JP4.5
  Top 0.406: IC2.9 54.11,33.07 R1.1
  Bottom 0.254: JP4.5 45.98,35.01 47,35.01 47.76,35.77 47.76,38.82 48.52,39.58 53.35,39.58 54.11,38.82 IC2.9
SCK
  Top 0.254: IC3.13 46.49,27.39 47.76,28.66 47.76,32.73 47.76,32.98 | 47.76,32.98 47.76,34 48.78,35.01 50.81,35.01 51.57,35.77 IC2.8 | JP4.3 47.76,32.98
SCL
  Top 0.305: IC2.22 79.51,51.27 80.27,50.51 90.43,50.51 91.45,49.49 JP2.1
  Top 0.61: JP2.1 91.45,45.68 91.96,45.17 R19.1
SDA
  Top 0.305: IC2.23 76.97,51.01 78.49,49.49 88.4,49.49 88.91,48.98 JP2.2
  Top 0.61: JP2.2 R20.1
SS
  Bottom 0.254: IC3.16 38.87,30.19 43.95,35.27 IC2.5
VCC
  Top 0.406: IC2.10 56.65,35.01 56.14,34.5 56.14,33 R1.2 56.14,32.94 56.14,31.71 54.87,30.44 JP4.2
  Top 0.61: C8.1 59.19,56.28 IC2.30 59.19,44.92 | 56.65,44.92 IC2.10 | JP3.1 91.45,51.52 94.24,48.73 94.24,43.9 92.53,42.19 R19.2 R20.2 88.91,41.87 88.65,42.12 85.86,42.12 83.07,44.92 59.19,44.92 | IC2.32 54.11,44.92 | 54.11,44.92 25.92,44.92 C2.+ | 54.11,44.92 56.65,44.92 | 56.65,44.92 59.19,44.92
  Top 0.813: IC1.1 14.49,38.82 15.76,37.55 24.39,37.55 | 24.39,37.55 C2.+ | 24.39,37.55 27.95,37.55 33.54,31.96 33.54,30.15 C7.1 33.79,29.89 IC3.18 33.79,23.07 31,20.28 31,14.69 28.2,11.9 21.6,11.9 20.11,13.39 IC4.5 20.07,14.93 20.07,16.72 22.65,19.3 IC4.3 22.65,26.4 C9.1
  Bottom 0.406: L1.2 13.47,48.69 13.47,45.93 14.49,44.92 IC1.1

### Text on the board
Top: IH_CON_h4
Bottom: IH_CON_h4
